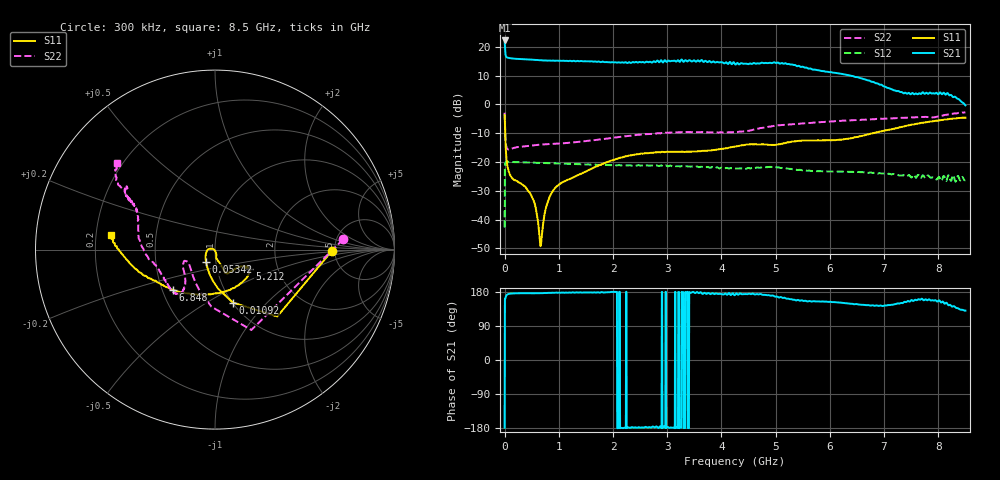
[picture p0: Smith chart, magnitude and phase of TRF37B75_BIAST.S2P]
!Agilent Technologies,E5071B,JP1KK00322,A.09.10
!Date: Mon Mar 03 16:09:12 2014
!Data & Calibration Information:
!Freq	S11:SOLT2(ON)	S21:SOLT2(ON)	S12:SOLT2(ON)	S22:SOLT2(ON)
# Hz S RI R 50
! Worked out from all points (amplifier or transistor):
!   1601 points, 300 kHz to 8.5 GHz, reference 50 ohm
!   highest |S21| = 22.2 dB at 300 kHz (marker M1)
!   |S21| within 3 dB of that: start of sweep to 8.742 MHz
!   unconditionally stable (mu >= 1): start of sweep to 912.2 kHz; 24.14 MHz to end of sweep
!   at 1.413 GHz: K = 1.17, MAG = 15.5 dB, |S12| = -20.8 dB
!   at 4.25 GHz: K = 1.32, MAG = 14.7 dB, |S12| = -22.2 dB
!   at 8.5 GHz: K = 3.05, MAG = 5.3 dB, |S12| = -26.3 dB
!   S11 on the Smith chart (normalised r, x): 300 kHz: 4.73, -0.12; 10.92 MHz: 1.01, -0.66; 53.42 MHz: 0.90, -0.12; 5.212 GHz: 1.43, -0.32; 6.848 GHz: 0.57, -0.28; 8.5 GHz: 0.26, +0.07
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300000  0.6513 -0.00718  -12.87 -0.2885  -0.00376 0.00622  0.7143 0.0569
1.092462e7  0.1003 -0.2954  -7.793 2.69  0.0861 0.0378  -0.0199 -0.318
5.342312e7  -0.0498 -0.0686  -6.429 0.7793  0.1003 0.0102  -0.1403 -0.0915
8.5297e7  -0.0525 -0.0383  -6.349 0.5967  0.1005 0.00772  -0.1486 -0.0732
1.649817e8  -0.0476 -0.0135  -6.211 0.4601  0.0996 0.00756  -0.1632 -0.0638
5.049697e8  -0.0239 0.00554  -5.962 0.3888  0.0959 0.0182  -0.1769 -0.0786
6.643391e8  -0.0027 -0.00217  -5.838 0.3653  0.0934 0.0237  -0.1785 -0.0912
8.927685e8  0.00751 -0.0307  -5.754 0.2695  0.0892 0.032  -0.1771 -0.1074
1.418687e9  0.0155 -0.0609  -5.662 0.2065  0.0764 0.0497  -0.1664 -0.1532
2.295219e9  0.0506 -0.1187  -5.398 -0.1576  0.0476 0.0737  -0.1751 -0.2236
2.837075e9  0.0665 -0.1321  -5.551 -0.052  0.0289 0.0802  -0.1966 -0.2473
3.602048e9  0.1065 -0.1109  -5.557 0.1896  -0.000637 0.0818  -0.2482 -0.2178
4.25015e9  0.1601 -0.0926  -4.937 0.7319  -0.0248 0.0734  -0.3076 -0.1216
4.696384e9  0.1735 -0.1017  -5.071 0.58  -0.0417 0.0676  -0.3823 -0.0307
4.993874e9  0.1742 -0.0938  -5.15 1.173  -0.0476 0.0657  -0.425 0.0612
5.211679e9  0.1912 -0.1058  -4.761 1.558  -0.0497 0.0595  -0.4283 0.125
5.668537e9  0.1546 -0.1785  -3.67 1.77  -0.056 0.0415  -0.4308 0.2065
6.847871e9  -0.2353 -0.2235  -1.876 1.374  -0.0644 0.00519  -0.4823 0.2834
7.086925e9  -0.3111 -0.1864  -1.567 1.108  -0.0627 -0.00328  -0.4873 0.2928
7.660655e9  -0.4642 -0.0873  -1.446 0.5533  -0.0515 -0.0169  -0.5032 0.3366
8.059078e9  -0.5349 -0.00181  -1.341 0.7115  -0.0378 -0.0282  -0.5279 0.3517
8.5e9  -0.5812 0.0839  -0.6222 0.7347  -0.0305 -0.0374  -0.5459 0.484
